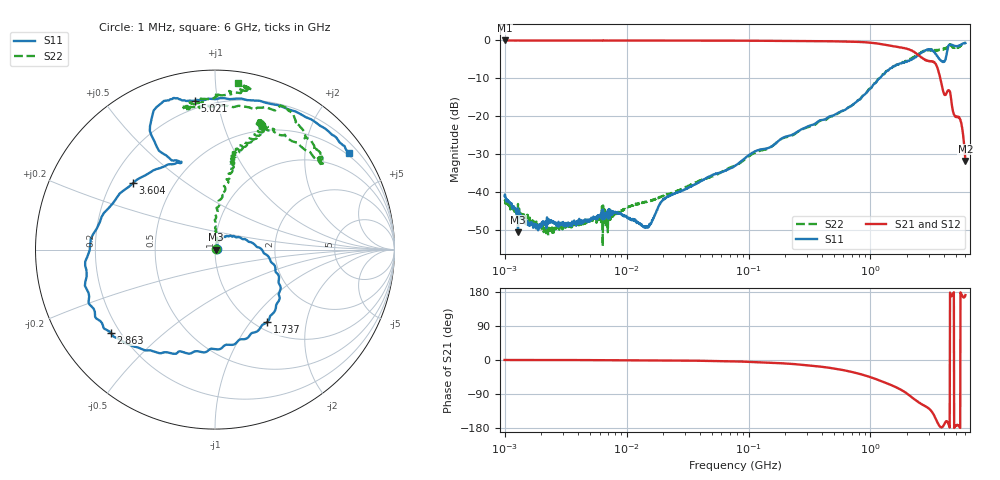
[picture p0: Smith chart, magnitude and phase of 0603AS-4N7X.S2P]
!s-Parameter Generated by FASTRON Sdn. Bhd.
!FASTRON P/N : 0603AS-4N7X
!Keysight Technologies: E5071C_MY46733604_B.14.02
!Date: Tue Nov 21 15:04:50 2023
!Version  :Rev01  Tue Nov 21 15:04:50 2023
!Data & Calibration Information:
!Freq  S11:SOLT2(ON)  S21:SOLT2(ON)  S12:SOLT2(ON)  S22:SOLT2(ON)
!PortZ  Port1:50+j0  Port2:50+j0
!When reading reference impedance value at option line is always used.
! Remarks : This data is being provided solely for informational purposes.
# Hz S dB R 50
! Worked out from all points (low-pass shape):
!   1601 points, 1 MHz to 6 GHz, reference 50 ohm
!   highest |S21| = -0.02 dB at 1.006 MHz (marker M1); lowest = -31.8 dB at 6 GHz (marker M2)
!   |S21| within 3 dB of the highest: start of sweep to 2.282 GHz
!   lowest |S11| = -50.6 dB at 1.288 MHz (marker M3), VSWR 1.01, Z = 50.3 - j0.0243 ohm
!   |S11| at or under -10 dB: start of sweep to 1.186 GHz
!   |S22| runs from -54.2 to -0.6 dB; largest |S21 - S12| = 0.0071
!   S11 on the Smith chart (normalised r, x): 1 MHz: 1.02, +0.01; 1.737 GHz: 1.14, -1.21; 2.863 GHz: 0.17, -0.34; 3.604 GHz: 0.29, +0.33; 5.021 GHz: 0.16, +0.86; 6 GHz: 0.43, +3.05
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1000000  -41.04 19.4  -0.03 0.1  -0.05 0.2  -42.34 24.4
1006392  -40.61 18.0  -0.02 0.1  -0.05 0.2  -42.12 20.7
1287650  -50.63 -4.7  -0.05 0.0  -0.06 0.1  -43.11 3.2
2178434  -48.33 37.4  -0.05 -0.1  -0.05 -0.1  -50.00 42.6
4277066  -48.19 33.9  -0.05 -0.2  -0.05 -0.2  -48.44 41.0
8079992  -45.19 43.6  -0.05 -0.4  -0.05 -0.4  -45.96 45.5
1.459489e7  -49.21 52.7  -0.04 -0.8  -0.06 -0.8  -42.50 39.4
1.823719e7  -43.86 53.2  -0.05 -1.0  -0.06 -0.9  -41.42 52.2
7.757876e7  -33.07 65.4  -0.08 -3.7  -0.08 -3.7  -33.01 67.3
3.307917e8  -22.29 56.3  -0.18 -14.9  -0.18 -14.9  -22.60 83.0
7.771452e8  -16.02 24.1  -0.39 -34.9  -0.40 -34.9  -15.94 90.1
1.414819e9  -7.70 -28.8  -1.33 -63.8  -1.34 -63.9  -7.73 78.0
1.737339e9  -6.07 -54.0  -1.87 -76.8  -1.87 -76.9  -6.00 78.3
2.291887e9  -4.53 -103.1  -3.08 -103.8  -3.09 -103.7  -4.32 72.9
2.863248e9  -2.59 -141.5  -5.23 -123.6  -5.20 -123.5  -2.74 68.4
3.239727e9  -2.79 -170.8  -5.51 -140.3  -5.47 -140.4  -2.74 69.7
3.604213e9  -4.62 140.9  -8.00 -169.3  -7.99 -169.7  -2.62 56.9
3.907951e9  -5.61 112.7  -12.86 -176.2  -12.87 -176.5  -2.39 40.5
4.19144e9  -3.97 119.5  -13.93 -161.3  -13.95 -161.6  -2.13 45.4
5.020705e9  -1.54 97.8  -20.20 -173.0  -20.24 -173.0  -1.92 97.8
5.524342e9  -1.11 64.4  -21.59 176.3  -21.59 176.5  -1.23 90.3
6e9  -0.71 35.7  -31.76 171.3  -31.74 171.3  -0.58 82.2
